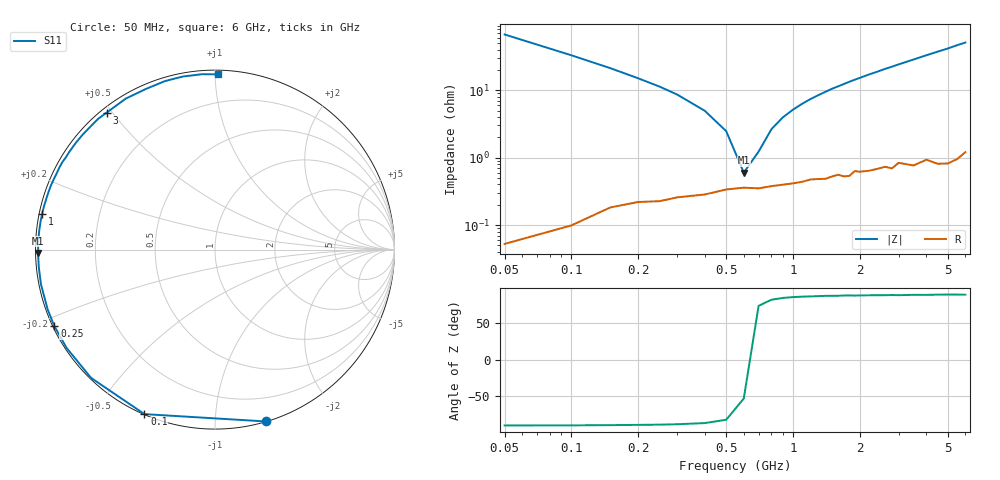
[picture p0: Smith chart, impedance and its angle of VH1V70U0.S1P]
! Infineon Technologies  Discrete & RF Semiconductors
! BB 814
! Si Tuning Diode in SOT23
! VR = 1.75 V
! S-Parameters:  July  1999
# GHz  S  MA  R  50
!  f  S11
! GHz  MAG  ANG
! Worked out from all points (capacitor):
!   34 points, 50 MHz to 6 GHz, reference 50 ohm
!   read as one part to ground: C = 47.1 pF near 50 MHz
!   lowest |Z| = 599 mohm at 600 MHz (marker M1)
!   series resonance near 628.9 MHz, so ESL is about 1.4 nH
!   S11 on the Smith chart (normalised r, x): 50 MHz: 0.00, -1.34; 100 MHz: 0.00, -0.66; 250 MHz: 0.00, -0.23; 1 GHz: 0.01, +0.10; 3 GHz: 0.02, +0.48; 6 GHz: 0.02, +1.02
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0.05  0.9992 -73.4
0.1  0.9972 -113.2
0.15  0.9938 -134.0
0.2  0.992 -146.5
0.25  0.9914 -154.5
0.3  0.99 -160.4
0.4  0.9888 -168.7
0.5  0.9866 -174.4
0.6  0.9858 -178.9
0.7  0.9861 177.3
0.8  0.985 174.0
0.9  0.9843 171.0
1  0.9837 168.3
1.2  0.9816 163.2
1.5  0.9801 156.3
1.6  0.979 154.3
1.8  0.9801 150.1
2  0.9776 146.2
2.2  0.9774 142.3
2.4  0.9765 138.8
2.8  0.9771 131.8
3  0.9732 128.4
3.5  0.9772 120.6
4  0.9744 113.2
4.5  0.9794 106.5
5  0.9808 100.5
5.5  0.9798 94.2
6  0.9766 89.0
